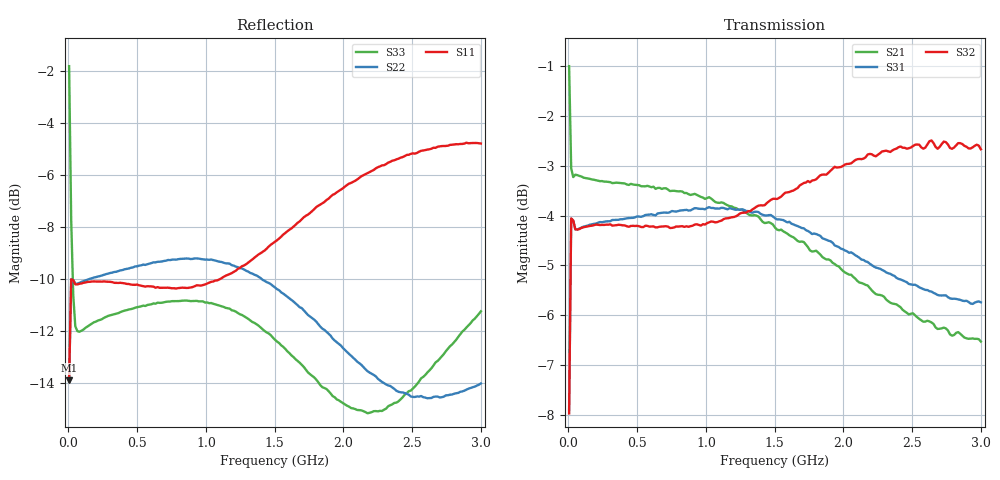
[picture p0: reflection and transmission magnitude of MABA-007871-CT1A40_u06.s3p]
#	MHz	S	RI	R	50
!FREQ	R1	I1	R2	I2	R3	I3
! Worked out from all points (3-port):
!   201 points, 5 MHz to 3 GHz, reference 50 ohm
!   strongest paths, dB at 5 MHz, 753.8 MHz, 1.502 GHz, 2.251 GHz, 3 GHz:
!     S32: -8.0, -4.2, -3.7, -2.8, -2.7
!     S31: -7.9, -3.9, -4.1, -5.1, -5.7
!     S21: -1.0, -3.5, -4.2, -5.6, -6.5
!   lowest |S11| = -13.9 dB at 5 MHz (marker M1), VSWR 1.51, Z = 60.8 + j20 ohm
!   |S11| at or under -10 dB: start of sweep to 1.102 GHz
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5  0.1263 0.158  0.8752 -0.1633  -0.2509 -0.3145
   0.8767 -0.1634  0.1233 0.1587  0.2489 0.3159
   -0.2509 -0.3145  0.2455 0.315  -0.5027 0.6352
19.975  0.3061 0.0781  0.6967 -0.1039  -0.6055 -0.1613
        0.6964 -0.1042  0.3034 0.0888  0.6027 0.1724
        -0.6055 -0.1613  0.6027 0.1723  0.2124 0.353
34.95  0.3142 0.0211  0.687 -0.0673  -0.6216 -0.0536
       0.6866 -0.0673  0.3127 0.0402  0.6196 0.0726
       -0.6216 -0.0536  0.6196 0.0727  0.2472 0.1606
154.75  0.3042 -0.0713  0.6747 -0.1293  -0.6125 0.0809
        0.6749 -0.1289  0.3164 0.00992  0.6164 0.00159
        -0.6125 0.0809  0.6161 0.00137  0.2519 0.0565
813.65  -0.000183 -0.3042  0.4094 -0.5305  -0.3912 0.5047
        0.4114 -0.5258  0.339 -0.0682  0.6079 -0.0996
        -0.3912 0.5047  0.6073 -0.1008  0.2866 -0.0177
1143.1  -0.2208 -0.233  0.1676 -0.628  -0.1707 0.6181
        0.1781 -0.6229  0.3162 -0.1223  0.6124 -0.1367
        -0.1707 0.6181  0.6117 -0.1374  0.2732 -0.0545
1502.5  -0.373 -0.00531  -0.1098 -0.5997  0.0934 0.6203
        -0.0955 -0.6063  0.2584 -0.1616  0.6302 -0.1927
        0.0934 0.6203  0.6269 -0.1938  0.2299 -0.0753
1876.875  -0.3437 0.2882  -0.3304 -0.4482  0.3132 0.5079
          -0.3238 -0.4692  0.1949 -0.1575  0.6435 -0.281
          0.3132 0.5079  0.6364 -0.2766  0.1871 -0.0537
2281.2  -0.1208 0.5084  -0.4472 -0.2241  0.4494 0.3284
        -0.4657 -0.2412  0.1579 -0.124  0.6194 -0.4051
        0.4494 0.3284  0.6145 -0.3977  0.1766 -0.00365
3000  0.364 0.4459  -0.4297 0.1467  0.5159 0.0198
      -0.4424 0.1631  0.1734 -0.0986  0.4506 -0.6011
      0.5159 0.0198  0.4458 -0.5853  0.2709 0.0427
